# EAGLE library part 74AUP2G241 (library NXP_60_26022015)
Low-power dual buffer/line driver; 3-state The 74AUP2G241 provides a dual non-inverting buffer/line driver with 3-state outputs. The 3-state outputs are controlled by the output enable inputs 1OE and 2OE. A HIGH level at pin 1OE causes output 1Y to assume a high-impedance OFF-state. A LOW level at pin 2OE causes output 2Y to assume a high-impedance OFF-state. Schmitt trigger action at all inputs makes the circuit tolerant to slower input rise and fall times across the entire VCC range from 0.8 V to 3.6 V. This device ensures a very low static and dynamic power consumption across the entire VCC range from 0.8 V to 3.6 V. This device is fully specified for partial power-down applications using IOFF. The IOFF circuitry disables the output, preventing the damaging backflow current through the device when it is powered down. This device has an input-disable feature, which allows floating input signals. The input 1A is disabled when the output enable input 1OE is HIGH. The input 2A is disabled when the output enable input 2OE is LOW. AAL Eindhoven MK
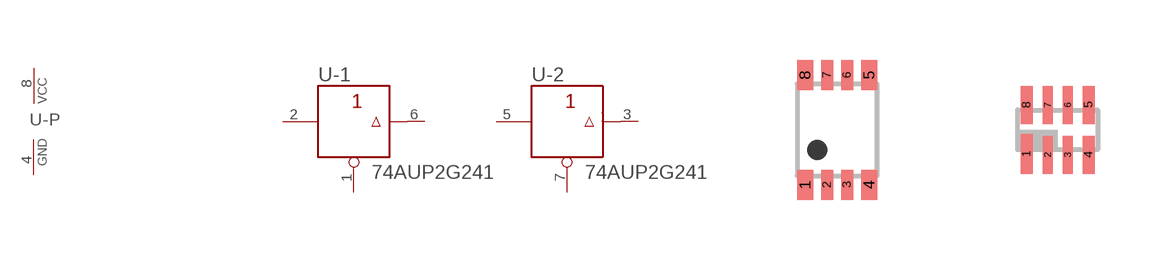
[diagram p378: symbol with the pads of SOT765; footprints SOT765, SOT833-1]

Designator prefix U; gates -P=PWRN -1=BUFFER_OE -2=BUFFER_OE

## 74AUP2G241DC  [SOT765]
1  -1:!OE  in
2  -1:A  in
3  -2:Y  out
4  -P:GND  pwr
5  -2:A  in
6  -1:Y  out
7  -2:!OE  in
8  -P:VCC  pwr

## 74AUP2G241GT  [SOT833-1]
Pads as for SOT765

## 74AUP2G241GF  [SOT1089-1]
Pads as for SOT765

## 74AUP2G241GD  [SOT996-2/3]
Pads as for SOT765

## 74AUP2G241GM  [SOT902-1/2/3]
Pads as for SOT765

## 74AUP2G241GS  [SOT1203]
Pads as for SOT765

## Footprint SOT765 (pad centres in mm)
SOT765 VSSOP8: plastic very thin shrink small outline package; 8 leads; body width 2.3 mm JEDEC: MO-187 IEC: -- JEITA: --
smd 0.4 x 0.75: 1 -0.8,-1.375; 4 0.8,-1.375; 5 0.8,1.375; 8 -0.8,1.375
smd 0.3 x 0.75: 2 -0.25,-1.375; 3 0.25,-1.375; 6 0.25,1.375; 7 -0.25,1.375

## Footprint SOT833-1 (pad centres in mm)
SOT833-1 XSON8: plastic extremely thin small outline package; no leads; 8 terminals; body 1 x 1.95 x 0.5 mm JEDEC: MO-252 IEC: -- JEITA: --
smd 0.3 x 1: 1 -0.775,-0.6
smd 0.25 x 0.95: 2 -0.25,-0.625; 3 0.25,-0.625; 6 0.25,0.625; 7 -0.25,0.625
smd 0.3 x 0.95: 4 0.775,-0.625; 5 0.775,0.625; 8 -0.775,0.625

## Footprint SOT1089-1 (pad centres in mm)
SOT1089-1 XSON8: plastic, extremely thin small outline package; no leads; 8 terminals; body 1 x 1.35 x 0.5 mm JEDEC: -- IEC: -- JEITA: --
smd 0.15 x 0.5: 1 -0.525,-0.35; 2 -0.175,-0.35; 3 0.175,-0.35; 4 0.525,-0.35; 5 0.525,0.35; 6 0.175,0.35; 7 -0.175,0.35; 8 -0.525,0.35

## Footprint SOT996-2/3 (pad centres in mm)
SOT996-2/3 XSON8U: plastic extremely thin small outline package; no leads;8 terminals; UTLP based; body 3 x 2 x 0.5 mm JEDEC: IEC: -- JEITA: --
smd 0.25 x 1.1: 1 -0.75,-1.45
smd 0.25 x 1: 2 -0.25,-1.5; 3 0.25,-1.5; 4 0.75,-1.5; 5 0.75,1.5; 6 0.25,1.5; 7 -0.25,1.5; 8 -0.75,1.5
